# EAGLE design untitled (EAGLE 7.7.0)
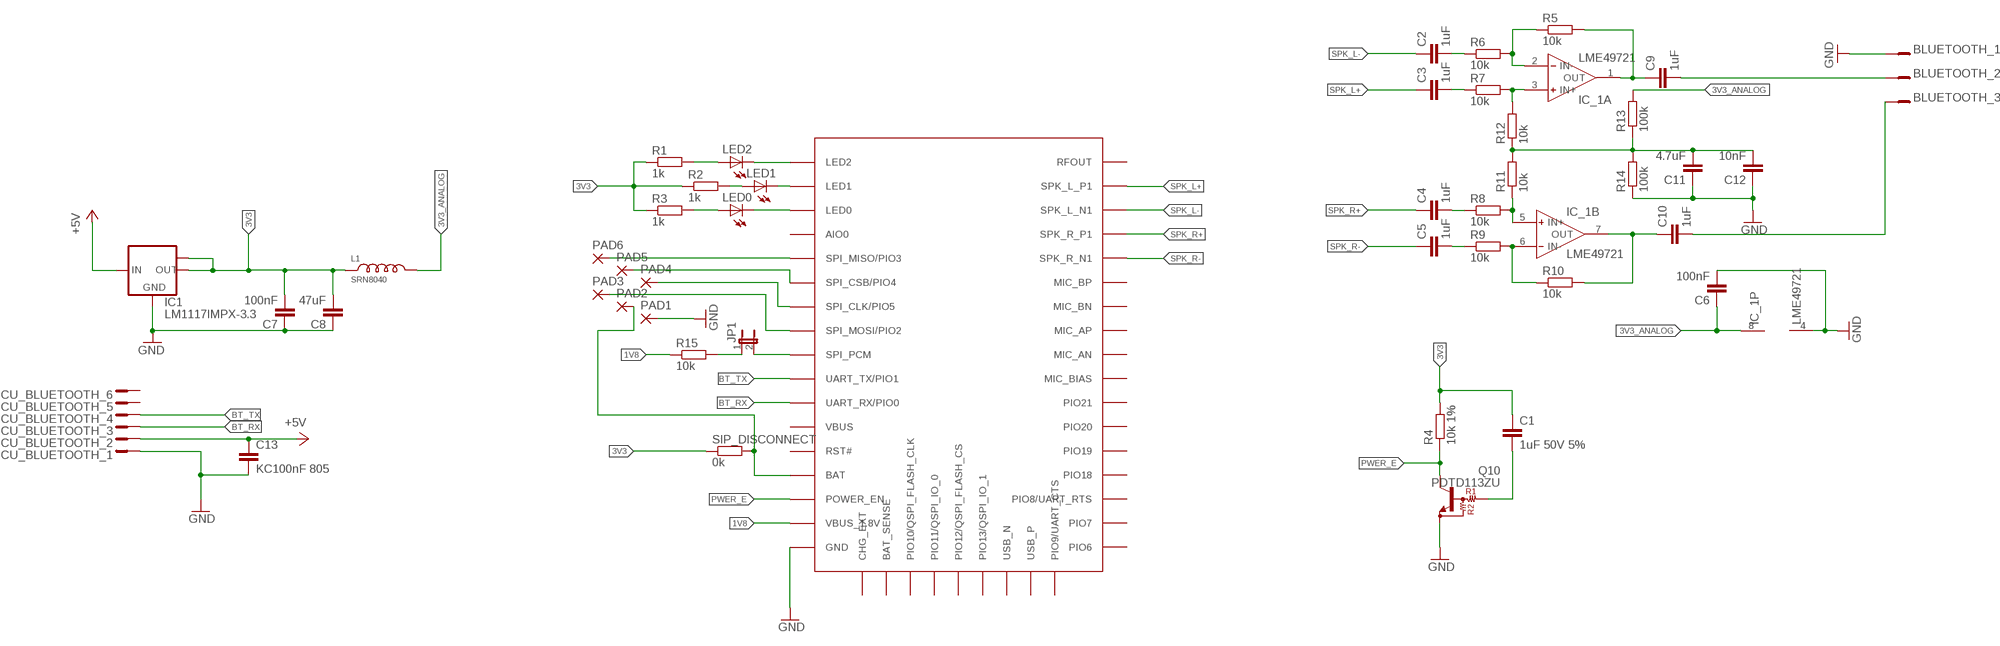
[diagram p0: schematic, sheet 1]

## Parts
BLUETOOTH  JST_3_PIN_B3B-PH-KS  [B3B-PH-KS]
C1  1uF 50V 5%  C-EUC0805  [C0805]
C2  1uF  C-EUC0805  [C0805]
C3  1uF  C-EUC0805  [C0805]
C4  1uF  C-EUC0805  [C0805]
C5  1uF  C-EUC0805  [C0805]
C6  100nF  C-EUC0805  [C0805]
C7  100nF  C-EUC0805  [C0805]
C8  47uF  C-EUC0805K  [C0805K]
C9  1uF  C-EUC0805  [C0805]
C10  1uF  C-EUC0805  [C0805]
C11  4.7uF  C-EUC0805  [C0805]
C12  10nF  C-EUC0805  [C0805]
C13  KC100nF 805  C-EUC0805  [C0805]
IC1  LM1117IMPX-3.3  [SOT223]
IC_1  LME49721  LME49721LME49721  [SOIC-8_NARROW]
JP1  JP1E  [JP1]
L1  SRN8040  [INDUCTOR_8X8]
LED0  LEDSMART-LED  [SMART-LED]
LED1  LEDSMART-LED  [SMART-LED]
LED2  LEDSMART-LED  [SMART-LED]
MCU_BLUETOOTH  JST_6_PIN_B6B-PH-KS  [B6B-PH-KS]
PAD1  SMD2  [SMD1,27-2,54]
PAD2  SMD2  [SMD1,27-2,54]
PAD3  SMD2  [SMD1,27-2,54]
PAD4  SMD2  [SMD1,27-2,54]
PAD5  SMD2  [SMD1,27-2,54]
PAD6  SMD2  [SMD1,27-2,54]
Q10  PDTD113ZU  [SOT-23]
R1  1k  R-EU_R0805  [R0805]
R2  1k  R-EU_R0805  [R0805]
R3  1k  R-EU_R0805  [R0805]
R4  10k 1%  R-EU_R0805  [R0805]
R5  10k  R-EU_R0805  [R0805]
R6  10k  R-EU_R0805  [R0805]
R7  10k  R-EU_R0805  [R0805]
R8  10k  R-EU_R0805  [R0805]
R9  10k  R-EU_R0805  [R0805]
R10  10k  R-EU_R0805  [R0805]
R11  10k  R-EU_R0805  [R0805]
R12  10k  R-EU_R0805  [R0805]
R13  100k  R-EU_R0805  [R0805]
R14  100k  R-EU_R0805  [R0805]
R15  10k  R-EU_R0805  [R0805]
SIP_DISCONNECT  0k  R-EU_R0805  [R0805]
U$4  F3188 - CSR8645 - GOOD  F3188  [F3188]

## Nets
1V8: R15.1 U$4.P$16(VBUS_1.8V)
3V3: C1.1 C7.2 C8.2 IC1.2(OUT) IC1.TAB(OUT1) L1.P$1 R1.1 R2.1 R3.1 R4.2 SIP_DISCONNECT.1
3V3_ANALOG: C6.1 IC_1.8(P:V+) L1.P$2 R13.2
+5V: C13.1 IC1.3(IN) MCU_BLUETOOTH.P$2
BT_AUDIO_L_OUT: BLUETOOTH.P$2 C9.2
BT_AUDIO_R_OUT: BLUETOOTH.P$3 C10.2
BT_RX: MCU_BLUETOOTH.P$3 U$4.P$11(UART_RX/PIO0)
BT_TX: MCU_BLUETOOTH.P$4 U$4.P$10(UART_TX/PIO1)
GND: BLUETOOTH.P$1 C6.2 C7.1 C8.1 C11.1 C12.1 C13.2 IC1.1(GND) IC_1.4(P:V-) MCU_BLUETOOTH.P$1 PAD1.1(P) Q10.2(E) R14.1 U$4.P$17(GND)
N$1: LED2.B(C) U$4.P$1(LED2)
N$2: LED1.B(C) U$4.P$2(LED1)
N$3: LED0.B(C) U$4.P$3(LED0)
N$4: LED2.A R1.2
N$5: LED1.A R2.2
N$6: LED0.A R3.2
N$7: IC_1.2(A:IN-) R5.1 R6.2
N$8: C2.2 R6.1
N$9: C1.2 Q10.1(B)
N$10: IC_1.3(A:IN+) R7.2 R12.2
N$11: C3.2 R7.1
N$12: IC_1.5(B:IN+) R8.2 R11.1
N$13: IC_1.6(B:IN-) R9.2 R10.1
N$14: C4.2 R8.1
N$15: C5.2 R9.1
N$16: PAD2.1(P) SIP_DISCONNECT.2 U$4.P$14(BAT)
N$20: C9.1 IC_1.1(A:OUT) R5.2
N$21: C10.1 IC_1.7(B:OUT) R10.2
N$23: C11.2 C12.2 R11.2 R12.1 R13.1 R14.2
N$25: PAD6.1(P) U$4.P$5(SPI_MISO/PIO3)
N$26: PAD5.1(P) U$4.P$6(SPI_CSB/PIO4)
N$27: PAD4.1(P) U$4.P$7(SPI_CLK/PIO5)
N$28: PAD3.1(P) U$4.P$8(SPI_MOSI/PIO2)
N$30: JP1.1 R15.2
PWER_E: Q10.3(C) R4.1 U$4.P$15(POWER_EN)
SPI_PCM: JP1.2 U$4.P$9(SPI_PCM)
SPK_L+: C3.1 U$4.P$42(SPK_L_P1)
SPK_L-: C2.1 U$4.P$41(SPK_L_N1)
SPK_R+: C4.1 U$4.P$40(SPK_R_P1)
SPK_R-: C5.1 U$4.P$39(SPK_R_N1)
Unconnected: MCU_BLUETOOTH.P$5 MCU_BLUETOOTH.P$6 U$4.P$4(AIO0) U$4.P$13(RST#) U$4.P$18(CHG_EXT) U$4.P$19(BAT_SENSE) U$4.P$20(PIO10/QSPI_FLASH_CLK) U$4.P$21(PIO11/QSPI_IO_0) U$4.P$22(PIO12/QSPI_FLASH_CS) U$4.P$23(PIO13/QSPI_IO_1) U$4.P$24(USB_N) U$4.P$25(USB_P) U$4.P$26(PIO9/UART_CTS) U$4.P$27(PIO6) U$4.P$28(PIO7) U$4.P$29(PIO8/UART_RTS) U$4.P$30(PIO18) U$4.P$31(PIO19) U$4.P$32(PIO20) U$4.P$33(PIO21) U$4.P$34(MIC_BIAS) U$4.P$35(MIC_AN) U$4.P$36(MIC_AP) U$4.P$37(MIC_BN) U$4.P$38(MIC_BP) U$4.P$43(RFOUT)

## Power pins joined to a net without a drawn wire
VBUS: U$4.P$12(VBUS)

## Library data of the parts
BLUETOOTH = conn-JST:JST_3_PIN_
C1 = resistor:C-EU: CAPACITOR, European symbol
C2-C13 = rcl:C-EU: CAPACITOR, European symbol
IC1 = lm1117:LM1117IMPX-*
IC_1 = lme49721:LME49721
JP1 = jumper:JP1E: JUMPER
L1 = ferrit_bear:SRN8040
LED0 LED1 LED2 = led:LED: LED
MCU_BLUETOOTH = conn-JST:JST_6_PIN_
PAD1-PAD6 = wirepad:SMD2: SMD PAD
Q10 = pre-bias-transistor:PDTD: Pre biase NPN transistor NPN Resistor-Equipped Transistor (RET) family in a very small SOT323 (SC-70) Surface-Mounted Device (SMD) plastic package. VCC = 50V Ic (max) = 500 mA; R1: 1 kOhm; R2: 10 kOhm
R1-R15 SIP_DISCONNECT = resistor:R-EU_: RESISTOR, European symbol
U$4 = f3188:F3188

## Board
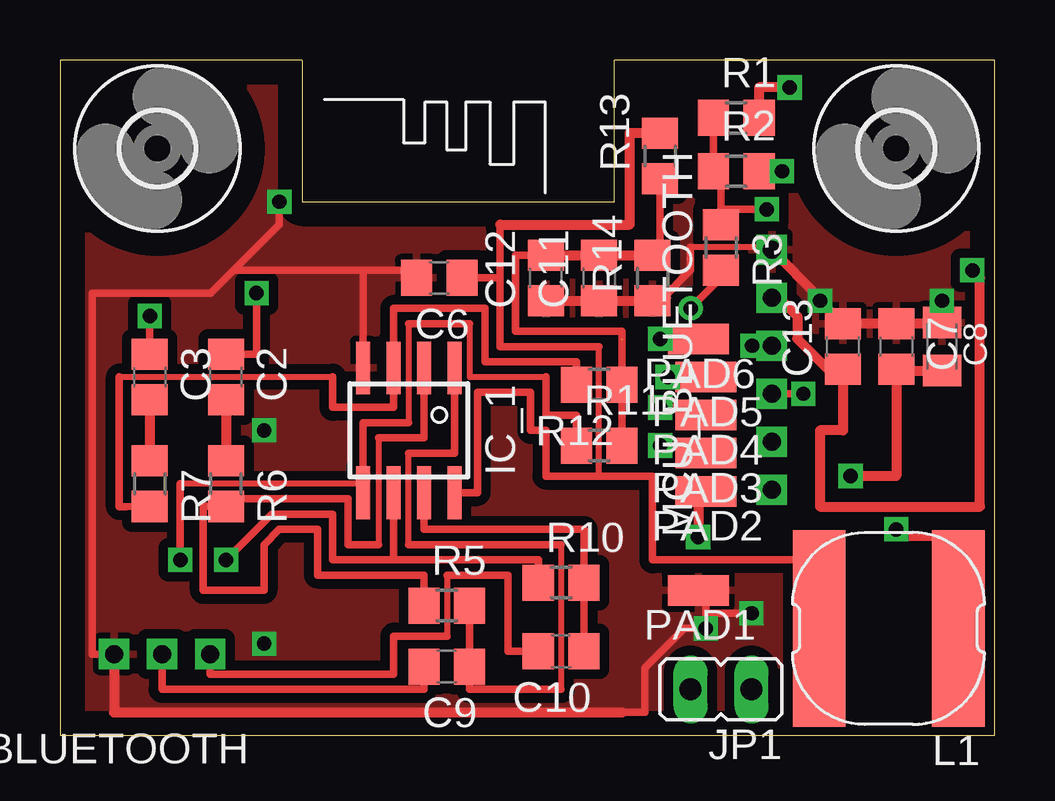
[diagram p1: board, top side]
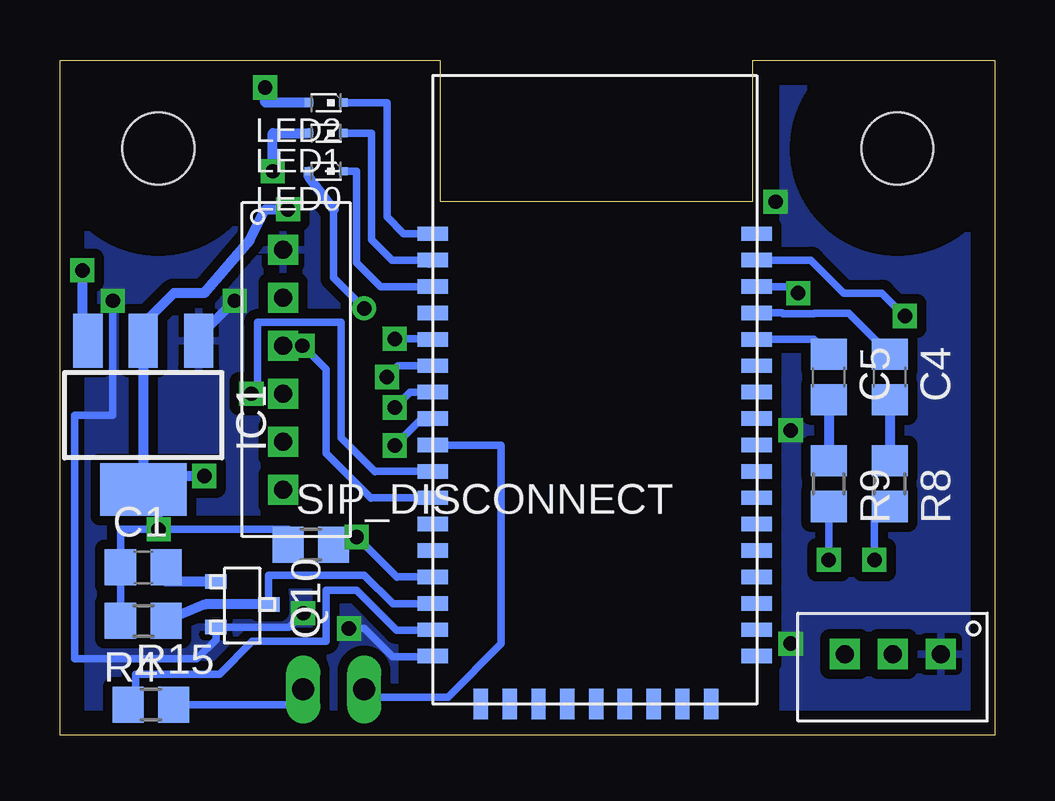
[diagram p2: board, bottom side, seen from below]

Size 38.97 x 28.13 mm. Coordinates in mm from the lower left corner, seen from the top.
Outline: 0,0 38.97,0 38.97,28.13 23.11,28.13 23.11,22.22 10.1,22.22 10.1,28.13 0,28.13 0,0
Copper layers (1*16): Top 0.035mm / dielectric 1.5mm / Bottom 0.035mm
Design rules "default": minimum track width 10mil, minimum drill 24mil, track to track 8mil, track to pad 8mil, pad to pad 8mil, via to via 8mil, smd to smd 8mil, copper to edge 40mil, drill to drill 8mil, minimum pad ring 10mil, minimum via ring 8mil, stop-mask expansion 4mil, vias tented up to drill 0mil, thermal gap 10mil

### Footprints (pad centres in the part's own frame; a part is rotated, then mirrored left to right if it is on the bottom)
B3B-PH-KS = drill 0.75 pad 1.2 square: P$1 -2,1.7; P$2 -4,1.7; P$3 -6,1.7
C0805 = smd 1.3 x 1.5: 1 -0.95,0; 2 0.95,0
C0805K = smd 1.3 x 1.6: 1 -1,0; 2 1,0
SOT223 = smd 1.219 x 2.235: 1 -2.311,-3.099; 2 0,-3.099; 3 2.311,-3.099 | smd 3.6 x 2.2: TAB 0,3.099
SOIC-8_NARROW = smd 0.6 x 2.2: 1 -1.905,-2.6; 2 -0.635,-2.6; 3 0.635,-2.6; 4 1.905,-2.6; 5 1.905,2.6; 6 0.635,2.6; 7 -0.635,2.6; 8 -1.905,2.6
JP1 = drill 0.914 long: 1 0,-1.27; 2 0,1.27
INDUCTOR_8X8 = smd 2.2 x 8.2: P$1 -2.9,0; P$2 2.9,0
SMART-LED = smd 0.35 x 0.35: A 0,0.725; B 0,-0.725
B6B-PH-KS = drill 0.75 pad 1.2 square: P$1 -2,1.7; P$2 -4,1.7; P$3 -6,1.7; P$4 -8,1.7; P$5 -10,1.7; P$6 -12,1.7
SMD1,27-2,54 = smd 1.27 x 2.54: 1 0,0
SOT-23 = smd 0.6 x 0.9: 1 -1,-1.1; 2 0.9,-1.1; 3 -0.05,1.1
R0805 = smd 1.3 x 1.5: 1 -0.95,0; 2 0.95,0
3,0 = hole 3: 0,0
F3188 = smd 1.27 x 0.6: P$1 -6.5,7.7; P$2 -6.5,6.6; P$3 -6.5,5.5; P$4 -6.5,4.4; P$5 -6.5,3.3; P$6 -6.5,2.2; P$7 -6.5,1.1; P$8 -6.5,0; P$9 -6.5,-1.1; P$10 -6.5,-2.2; P$11 -6.5,-3.3; P$12 -6.5,-4.4; P$13 -6.5,-5.5; P$14 -6.5,-6.6; P$15 -6.5,-7.7; P$16 -6.5,-8.8; P$17 -6.5,-9.9; P$27 7,-9.9; P$28 7,-8.8; P$29 7,-7.7; P$30 7,-6.6; P$31 7,-5.5; P$32 7,-4.4; P$33 7,-3.3; P$34 7,-2.2; P$35 7,-1.1; P$36 7,0; P$37 7,1.1; P$38 7,2.2; P$39 7,3.3; P$40 7,4.4; P$41 7,5.5; P$42 7,6.6; P$43 7,7.7 | smd 0.6 x 1.27: P$18 -4.5,-11.9; P$19 -3.3,-11.9; P$20 -2.1,-11.9; P$21 -0.9,-11.9; P$22 0.3,-11.9; P$23 1.5,-11.9; P$24 2.7,-11.9; P$25 3.9,-11.9; P$26 5.1,-11.9

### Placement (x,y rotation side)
BLUETOOTH  0.25,5.08 180 top
C1  35.5,6.98 0 bottom
C2  6.92,14.92 270 top
C3  3.75,14.92 270 top
C4  4.38,14.92 270 bottom
C5  6.92,14.92 270 bottom
C6  15.81,19.05 180 top
C7  34.86,16.19 270 top
C8  36.77,16.19 270 top
C9  16.13,2.86 180 top
C10  20.89,3.49 180 top
C11  22.48,19.05 90 top
C12  20.26,19.05 90 top
C13  32.64,16.19 90 top
IC1  35.5,13.33 180 bottom
IC_1  14.54,12.7 180 top
JP1  27.56,1.9 90 top
L1  34.54,4.44 180 top
LED0  27.88,23.5 90 bottom
LED1  27.88,25.08 90 bottom
LED2  27.88,26.35 90 bottom
MCU_BLUETOOTH  31.37,22.22 90 top
PAD1  26.61,6.03 90 top
PAD2  26.92,10.16 90 top
PAD3  26.92,11.75 90 top
PAD4  26.92,13.33 90 top
PAD5  26.92,14.92 90 top
PAD6  26.61,16.51 90 top
Q10  31.37,5.4 270 bottom
R1  28.19,25.72 0 top
R2  28.19,23.5 0 top
R3  27.56,20.32 270 top
R4  35.5,4.76 180 bottom
R5  16.13,5.4 0 top
R6  6.92,10.48 270 top
R7  3.75,10.48 270 top
R8  4.38,10.48 270 bottom
R9  6.92,10.48 270 bottom
R10  20.89,6.35 0 top
R11  22.48,12.06 0 top
R12  22.48,14.6 180 top
R13  25.02,24.13 90 top
R14  24.7,19.05 90 top
R15  35.18,1.27 0 bottom
SIP_DISCONNECT  28.51,7.94 0 bottom
U$2  [3,0]  4.06,24.45 0 top
U$3  [3,0]  34.86,24.45 0 top
U$4  16.92,13.19 0 bottom

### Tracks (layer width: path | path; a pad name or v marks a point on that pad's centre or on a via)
1V8
  Bottom 0.305: R15.1 35.81,1.58 35.81,2.54 32.32,2.54 30.95,3.91 27.88,3.91 27.88,6.03 26.61,6.03 24.94,4.37 23.44,4.37 U$4.P$16
3V3  (via drill 0.6)
  Top 0.305: L1.P$1 37.44,8.25 34.86,8.25 v34.86,8.57 | R1.1 R2.1 | 27.56,23.49 27.56,21.91 | v29.46,21.91 27.56,21.91 | 27.56,21.91 R3.1
  Top 0.406: 34.86,15.19 C8.2 | C7.2 34.86,15.19 | 34.86,15.19 34.86,10.79 v32.96,10.79 | R2.1 27.56,23.49
  Bottom 0.305: C1.1 R4.2 36.45,8.57 v34.86,8.57 | v34.86,8.57 34.86,10.24 IC1.TAB | SIP_DISCONNECT.1 29.46,8.57 v34.86,8.57
  Bottom 0.406: IC1.2 35.5,10.79 | v32.96,10.79 35.5,10.79 | 35.5,10.79 IC1.TAB | IC1.2 35.25,16.43 | IC1.2 35.5,17.14 34.23,18.41 32.96,18.41 31.05,20.64 30.41,21.91 30.1,21.91 v29.46,21.91
3V3_ANALOG
  Top 0.254: 22.48,10.79 22.48,16.19
  Top 0.305: 31.69,3.81 31.64,3.85 L1.P$2 31.69,4.44 31.69,7.3 24.7,7.3 24.7,10.79 22.48,10.79 20.26,10.79 20.26,12.7 19.62,12.7 19.62,14.29 17.4,14.29 17.4,10.1 IC_1.8 | 22.48,16.19 18.35,16.19 18.35,19.05 | 18.35,19.05 18.35,21.27 | C6.1 18.35,19.05
  Top 0.406: R13.2 23.75,25.08 23.75,21.27 18.35,21.27
+5V  (via drill 0.6)
  Top 0.406: MCU_BLUETOOTH.P$2 29.97,18.22 30.73,17.46 30.73,16.52 32.02,15.24 C13.1 32.64,12.7 31.69,12.7 31.69,9.52 38.35,9.52 38.35,19.05 v38.04,19.37
  Bottom 0.406: v38.04,19.37 38.04,16.43 IC1.3
BT_AUDIO_L_OUT
  Top 0.305: BLUETOOTH.P$2 4.25,1.9 15.18,1.9 C9.2
BT_AUDIO_R_OUT
  Top 0.254: 16.13,6.67 16.13,4.13
  Top 0.305: 16.13,6.67 18.67,6.67 18.67,3.49 C10.2 | 16.13,4.13 13.91,4.13 13.91,2.54 6.25,2.54 BLUETOOTH.P$3 6.25,2.86
BT_RX  (via drill 0.6)
  Top 0.305: v28.86,16.22 MCU_BLUETOOTH.P$3
  Bottom 0.305: v28.86,16.22 27.88,15.24 27.88,11.75 26,9.87 25.98,9.89 U$4.P$11
BT_TX  (via drill 0.6)
  Top 0.305: v30.99,14.22 MCU_BLUETOOTH.P$4
  Bottom 0.305: v30.99,14.22 30.73,14.29 30.73,17.2 27.24,17.2 27.24,12.38 26.29,11.43 | 25.83,10.97 26.29,11.43 | U$4.P$10 25.85,10.99 26.29,11.43
GND  (via drill 0.6)
  Top 0.254: 29.57,20.32 26.29,20.32
  Top 0.305: v36.77,18.1 C8.1 | MCU_BLUETOOTH.P$1 29.57,20.32 | 27.24,5.08 v28.83,5.08 26.92,5.08 | 26.92,5.08 v26.92,4.44 26.03,4.44 24.38,2.8 24.38,0.95 23.43,0.95 | 12.64,19.37 IC_1.4 | BLUETOOTH.P$1 1.35,3.38 1.35,18.41 6.29,18.41 7.24,19.37 | 7.24,19.37 12.64,19.37 | R14.1 25.02,18.1 26.29,19.37 26.29,20.32 | PAD1.1 26.92,5.71 26.92,5.08 | C6.2 14.54,19.37 12.64,19.37 | 7.24,19.37 9.14,21.27 v9.14,22.22
  Top 0.406: C12.1 C11.1 R14.1 | BLUETOOTH.P$1 2.25,0.95 23.43,0.95 | MCU_BLUETOOTH.P$1 31.69,18.21 v31.69,18.1 C13.2 C7.1 36.72,17.14 C8.1
  Bottom 0.305: v36.77,18.1 36.77,13.33 38.35,13.33 38.35,3.17 33.27,3.17 32.47,3.98 Q10.2 29.41,4.5 v28.83,5.08 | v26.92,4.44 26.29,4.44 25.11,3.27 23.44,3.27 arc-90 U$4.P$17
  Bottom 0.406: IC1.1 33.18,16.6 v31.69,18.1
  other vias: 8.51,3.81 8.51,12.7
  pour Top (isolate 0.406): -0.38,-1.27 -0.38,27.94 10.41,27.94 10.41,22.86 23.75,22.86 23.75,27.94 40.26,27.94 40.26,-1.27
  pour Bottom (isolate 0.406): -1.65,-1.27 -1.65,27.94 8.83,27.94 8.83,-0.32 25.02,-0.32 25.02,27.94 40.26,27.94 40.26,-1.27
N$1
  Bottom 0.305: LED2.B 25.34,26.35 25.34,21.59 24.64,20.89 U$4.P$1
N$2
  Bottom 0.305: LED1.B 25.97,25.08 25.97,20.64 25.12,19.79 U$4.P$2 arc-90 23.58,19.63
N$3
  Bottom 0.305: LED0.B 26.61,23.5 26.61,19.68 25.61,18.69 U$4.P$3
N$4  (via drill 0.6)
  Top 0.406: v30.42,26.99 29.14,26.99 R1.2
  Bottom 0.406: LED2.A 30.42,26.35 v30.42,26.99
N$5  (via drill 0.6)
  Top 0.406: R2.2 v30.1,23.5
  Bottom 0.406: v30.1,23.5 30.1,25.08 LED1.A
N$6  (via drill 0.6)
  Top 0.305: v26.29,17.78 27.56,19.05 R3.2
  Bottom 0.305: 27.56,21.91 27.56,19.05 v26.29,17.78
  Bottom 0.406: 27.56,21.91 28.6,23.27 LED0.A
N$7
  Top 0.254: 13.27,12.38 13.27,7.94
  Top 0.305: IC_1.2 15.18,12.38 13.27,12.38 | 13.27,7.94 12,7.94 12,9.84 6.92,9.84 R6.2 | 7.24,9.84 R6.2 | R5.1 15.18,6.67 10.73,6.67 10.73,8.57 9.14,8.57 8.51,7.94 8.51,6.03 5.97,6.03 5.97,9.53 R6.2
N$8
  Top 0.406: C2.2 R6.1
N$9
  Bottom 0.406: Q10.1 34.55,6.4 C1.2
N$10
  Top 0.254: 2.48,14.92 11.37,14.92
  Top 0.305: R7.2 2.79,9.52 2.48,9.52 2.48,14.92 | 11.37,14.92 11.37,13.65 13.91,13.65 IC_1.3 13.91,17.78 17.72,17.78 17.72,15.56 21.53,15.56 R12.2
N$11
  Top 0.406: C3.2 R7.1
N$12  (via drill 0.6)
  Top 0.254: 14.54,17.14 14.54,13.02 | 12.64,10.48 5.02,10.48 | 17.08,17.14 17.08,14.92 20.26,14.92
  Top 0.305: 17.08,17.14 14.54,17.14 | 14.54,13.02 12.64,13.02 IC_1.5 12.64,10.48 | 5.02,10.48 v5.02,7.3 | 20.26,14.92 20.26,13.33 21.53,13.33 R11.1
  Bottom 0.305: R8.2 5.02,8.89 v5.02,7.3
N$13  (via drill 0.6)
  Top 0.305: 13.91,7.3 IC_1.6 | R10.1 19.94,7.3 13.91,7.3 | v6.92,7.3 8.83,9.21 11.37,9.21 11.37,7.3 13.91,7.3
  Bottom 0.305: v6.92,7.3 R9.2
N$14
  Bottom 0.406: C4.2 R8.1
N$15
  Bottom 0.406: C5.2 R9.1
N$16  (via drill 0.6)
  Top 0.406: 26.61,10.16 PAD2.1 26.61,10.16 v26.61,8.25
  Bottom 0.305: 26.29,7.94 v26.61,8.25 | SIP_DISCONNECT.2 26.29,7.94 | 26.29,7.94 26.13,7.78 24.92,6.57 24.9,6.59 U$4.P$14
N$20
  Top 0.254: 20.89,7.94 20.89,1.9 | 14.54,7.94 14.54,11.75
  Top 0.305: R5.2 C9.1 17.08,1.9 20.89,1.9 | 20.89,7.94 14.54,7.94 | 14.54,11.75 16.45,11.75 IC_1.1
N$21
  Top 0.305: C10.1 R10.2 21.84,8.57 15.18,8.57 IC_1.7
N$23
  Top 0.305: C12.2 18.99,20 18.99,16.83 23.43,16.83 R12.1 R11.2 | R14.2 25.02,20 R13.1
  Top 0.406: R14.2 C11.2 C12.2
N$25  (via drill 0.6)  (1 unrouted)
  Top 0.305: v25.02,16.51 PAD6.1
  Bottom 0.305: 23.46,16.51 v25.02,16.51
N$26  (via drill 0.6)
  Top 0.305: v25.34,14.92 PAD5.1
  Bottom 0.305: 24.89,15.37 25.02,15.24 | 25.02,15.24 v25.34,14.92 | U$4.P$6 24.87,15.39 25.02,15.24
N$27  (via drill 0.6)
  Top 0.305: v25.02,13.65 25.65,13.65 PAD4.1
  Bottom 0.305: U$4.P$7 24.38,14.29 v25.02,13.65
N$28  (via drill 0.6)
  Top 0.305: v25.02,12.06 26.61,12.06 PAD3.1
  Bottom 0.305: 23.91,13.17 24.07,13.02 | 24.07,13.02 v25.02,12.06 | U$4.P$8 arc90 23.59,13.02 24.07,13.02
N$30
  Bottom 0.305: JP1.1 29.46,1.27 R15.2
PWER_E
  Bottom 0.305: Q10.3 30.27,6.67 26.29,6.67 25.09,5.47 23.44,5.47 U$4.P$15
  Bottom 0.406: R4.1 32.91,5.45 Q10.3 30.27,5.4
SPI_PCM
  Bottom 0.305: JP1.2 26.29,1.59 22.8,1.59 20.57,3.81 20.57,12.07 23.4,12.07 arc90 U$4.P$9
SPK_L+  (via drill 0.6)
  Top 0.305: v3.75,17.46 C3.1
  Bottom 0.305: v3.75,17.46 4.7,18.41 6.29,18.41 7.66,19.79 U$4.P$42
SPK_L-  (via drill 0.6)
  Top 0.305: C2.1 8.19,15.87 v8.19,18.41
  Bottom 0.305: 8.19,18.37 v8.19,18.41 8.19,18.67 8.21,18.69 U$4.P$41
SPK_R+
  Bottom 0.305: C4.1 6.08,17.57 7.53,17.57 7.54,17.56 8.84,17.56 8.88,17.59 U$4.P$40
SPK_R-
  Bottom 0.305: 7.24,16.15 C5.1 7.4,16.35 | 7.52,16.47 7.4,16.35 | U$4.P$39 7.54,16.49 7.4,16.35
